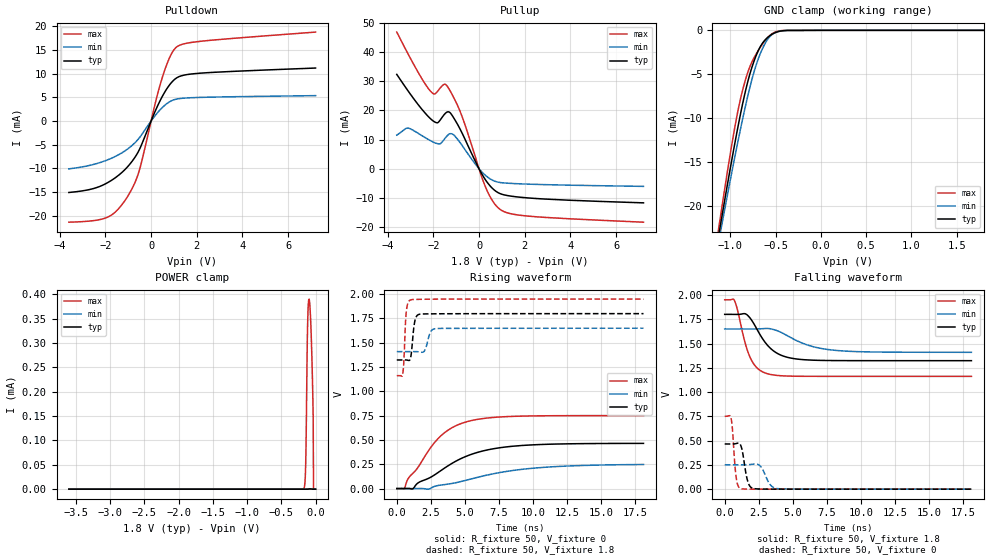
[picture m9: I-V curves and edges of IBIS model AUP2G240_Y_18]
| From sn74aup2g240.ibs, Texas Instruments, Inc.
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[Model]   AUP2G240_Y_18
Model_type  3-state
Enable   Active-Low
Vref =   0
Rref =   1E6
Cref =   30p
Vmeas =   0.9
| variable   typ   min   max
C_comp   2.13pF   1.92pF   2.45pF
| C_pullup   2.97pF   2.11pF   3.72pF
| C_pulldown   2.49pF   2.23pF   2.87pF
| C_tri-state   2.13pF   1.92pF   2.45pF
[Temperature Range]   40   100   -40
| Ambient temperature   25   85   -40
[Voltage range]   1.8   1.65   1.95
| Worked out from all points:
|   slope of the pulldown table from 0 to 0.27 V, typ, clamps not added: 88.7 ohm
|   slope of the pullup table from 0 to 0.27 V, typ, clamps not added: 73.8 ohm
|   GND clamp passes 1 mA (typ) near -0.61 V on its own axis
|   rising waveform, R_fixture 50, V_fixture 0: 20-80 % time 3.79ns typ, 5.28ns min, 2.63ns max; typ from 0 V to 0.465 V
|   falling waveform, R_fixture 50, V_fixture 1.8: 20-80 % time 1.5ns typ, 2.46ns min, 971ps max; typ from 1.8 V to 1.32 V
|   rising waveform, R_fixture 50, V_fixture 1.8: 20-80 % time 211ps typ, 289ps min, 156ps max; typ from 1.32 V to 1.8 V
|   falling waveform, R_fixture 50, V_fixture 0: 20-80 % time 345ps typ, 523ps min, 238ps max; typ from 0.465 V to 0 V
[GND Clamp]
| AUP2G240_Y_18
|   Voltage   I(typ)   I(min)   I(max)
-3.6V     -191.7mA   -177.9mA   -208.5mA
-1.145V   -24.23mA   -24.86mA   -23.52mA
-1.12V    -22.7mA    -23.46mA   -21.81mA
-1.095V   -21.18mA   -22.08mA   -20.12mA
-945mV    -12.48mA   -14.04mA   -10.63mA
-840mV    -7.167mA   -8.879mA   -5.824mA
-770mV    -4.441mA   -5.866mA   -3.761mA
-695mV    -2.366mA   -3.314mA   -2.326mA
-615mV    -1.069mA   -1.454mA   -1.136mA
-540mV    -445.1uA   -476.9uA   -389.8uA
-375mV    -14.91uA   -17.49uA   -5.064uA
1.8V      156.7pA    6.089nA    32.78pA
[POWER Clamp]
| AUP2G240_Y_18
|   Voltage   I(typ)   I(min)   I(max)
-3.6V     1.629nA    3.068nA    591.4pA
-175mV    1.002nA    3.126nA    789.8nA
-155mV    3.029nA    5.176nA    13.52uA
-145mV    6.961nA    7.247nA    46.67uA
-120mV    71.57nA    17.43nA    310.6uA
-115mV    111nA      20.14nA    345.5uA
-95mV     427.4nA    26.86nA    390.2uA
-70mV     520.6nA    18.99nA    340.4uA
-45mV     60.11nA    5.162nA    220.7uA
-35mV     403.6pA    2.686nA    149.2uA
-30mV     342.7pA    1.953nA    43.02pA
0V        0A         0A         0A
[Pulldown]
| AUP2G240_Y_18
|   Voltage   I(typ)   I(min)   I(max)
-3.6V     -15.09mA   -10.1mA    -21.36mA
-1.91V    -13.03mA   -8.209mA   -20.31mA
-1.48V    -11.66mA   -7.264mA   -18.79mA
-1.025V   -9.634mA   -5.896mA   -15.9mA
-725mV    -7.781mA   -4.672mA   -13.18mA
-520mV    -6.099mA   -3.589mA   -10.49mA
205mV     2.352mA    1.308mA    4.202mA
545mV     5.664mA    3.086mA    10.01mA
855mV     7.912mA    4.18mA     13.84mA
1.115V    9.087mA    4.628mA    15.61mA
2.18V     10.1mA     4.986mA    16.83mA
7.2V      11.18mA    5.355mA    18.77mA
[Pullup]
| AUP2G240_Y_18
|   Voltage   I(typ)   I(min)   I(max)
-3.6V     32.35mA    11.53mA    46.85mA
-3.1V     26.62mA    13.94mA    39.28mA
-2.125V   17.16mA    9.635mA    26.61mA
-1.94V    16.04mA    8.926mA    25.63mA
-1.7V     16.71mA    8.579mA    27.68mA
-1.485V   18.91mA    10.46mA    28.96mA
-1.28V    19.3mA     11.97mA    26.9mA
-740mV    12.21mA    7.998mA    17.86mA
290mV     -3.896mA   -2.327mA   -6.363mA
905mV     -8.461mA   -4.699mA   -13.83mA
2.165V    -10.01mA   -5.277mA   -16.25mA
7.2V      -11.69mA   -6.041mA   -18.32mA
[Ramp]
| AUP2G240_Y_18
| variable   typ   min   max
dV/dt_r   0.28/3.84E-09   0.15/5.44E-09   0.45/2.64E-09
dV/dt_f   0.29/1.51E-09   0.15/2.48E-09   0.48/9.76E-10
R_load = 50
[Rising Waveform]
| AUP2G240_Y_18
R_fixture =   50
C_fixture =   0
L_fixture =   0
V_fixture =   0
V_fixture_min = 0
V_fixture_max = 0
|   Time   V(typ)   V(min)   V(max)
0s        6.973nV    25.3nV     613.1pV
569ps     5.851uV    -5.08uV    2.822mV
889ps     734uV      -24.58uV   113.4mV
1.161ns   -3.328mV   -1.757uV   154.2mV
2.341ns   106.1mV    -5.639mV   392.7mV
3.125ns   174.4mV    33.73mV    527.8mV
5.041ns   329.1mV    84.11mV    683.9mV
6.929ns   405.6mV    147.9mV    730mV
9.181ns   443.2mV    197.8mV    745.5mV
18.09ns   465mV      247.7mV    750.8mV
[Falling Waveform]
| AUP2G240_Y_18
R_fixture =   50
C_fixture =   0
L_fixture =   0
V_fixture =   1.8
V_fixture_min = 1.65
V_fixture_max = 1.95
|   Time   V(typ)   V(min)   V(max)
0s        1.8V       1.65V      1.95V
713ps     1.8V       1.65V      1.943V
1.509ns   1.806V     1.65V      1.501V
1.869ns   1.761V     1.65V      1.355V
2.405ns   1.637V     1.65V      1.244V
3.065ns   1.494V     1.655V     1.192V
4.545ns   1.36V      1.584V     1.165V
6.125ns   1.331V     1.482V     1.162V
7.769ns   1.325V     1.435V     1.162V
18.09ns   1.323V     1.409V     1.162V
[Rising Waveform]
| AUP2G240_Y_18
R_fixture =   50
C_fixture =   0
L_fixture =   0
V_fixture =   1.8
V_fixture_min = 1.65
V_fixture_max = 1.95
|   Time   V(typ)   V(min)   V(max)
0s        1.323V     1.409V     1.162V
421ps     1.323V     1.409V     1.171V
501ps     1.323V     1.409V     1.266V
629ps     1.323V     1.409V     1.683V
701ps     1.323V     1.409V     1.825V
1.037ns   1.362V     1.41V      1.942V
1.325ns   1.724V     1.41V      1.946V
1.689ns   1.794V     1.405V     1.947V
2.869ns   1.798V     1.646V     1.949V
18.09ns   1.8V       1.65V      1.95V
[Falling Waveform]
| AUP2G240_Y_18
R_fixture =   50
C_fixture =   0
L_fixture =   0
V_fixture =   0
V_fixture_min = 0
V_fixture_max = 0
|   Time   V(typ)   V(min)   V(max)
0s        465.4mV    251mV      750.9mV
489ps     465mV      251mV      715.9mV
833ps     469.4mV    250.8mV    130.9mV
1.173ns   451.9mV    250.6mV    5.975mV
1.685ns   82.86mV    252.1mV    839.8uV
2.117ns   6.701mV    257.8mV    315.5uV
2.605ns   1.64mV     238.5mV    134.3uV
3.313ns   483.1uV    50.23mV    43.36uV
3.873ns   235.4uV    5.672mV    18.02uV
18.09ns   42.39nV    254.5nV    9.819nV
